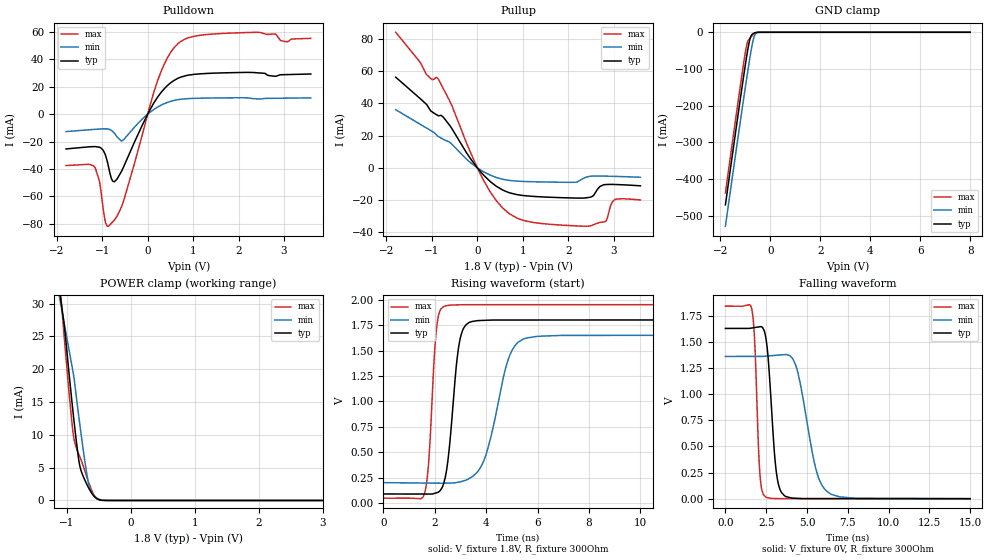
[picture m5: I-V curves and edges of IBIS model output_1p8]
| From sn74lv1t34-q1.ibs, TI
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[Model]   output_1p8
Model_type   Output
Polarity   Non-Inverting
Vmeas = 0.9
Vref = 0.9
Cref = 15pF
Rref = 100000
|   typ   min   max
C_comp   4.947pF   4.835pF   5.043pF
[Voltage Range]   1.8   1.65   1.95
[Temperature Range]   27   125   -40
[Pullup Reference]   1.8   1.65   1.95
[Pulldown Reference]   0   0   0
[Power Clamp Reference]   1.8   1.65   1.95
[GND Clamp Reference]   0   0   0
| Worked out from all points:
|   slope of the pulldown table from 0 to 0.27 V, typ, clamps not added: 18.4 ohm
|   slope of the pullup table from 0 to 0.27 V, typ, clamps not added: 33.4 ohm
|   GND clamp passes 1 mA (typ) near -0.59 V on its own axis
|   POWER clamp passes 1 mA (typ) near -0.60 V on its own axis
|   rising waveform, V_fixture 1.8V, R_fixture 300Ohm: 20-80 % time 371ps typ, 784ps min, 246ps max; typ from 0.092 V to 1.8 V
|   falling waveform, V_fixture 0V, R_fixture 300Ohm: 20-80 % time 430ps typ, 961ps min, 261ps max; typ from 1.63 V to 0 V
[Pulldown]
|   Voltage   I(typ)   I(min)   I(max)
-1.796V   -25.37mA   -12.71mA   -37.49mA
-1.156V   -23.66mA   -11.08mA   -39.01mA
-1.062V   -24.1mA    -10.87mA   -48.82mA
-925mV    -30.32mA   -10.72mA   -79.27mA
-767.5mV  -48.96mA   -12.71mA   -78.42mA
-557.5mV  -40.37mA   -19.33mA   -65.89mA
282.5mV   15.25mA    6.303mA    30mA
576.5mV   24.48mA    9.931mA    48.22mA
839mV     28.01mA    11.17mA    54.92mA
2.414V    30.08mA    11.11mA    59.61mA
3.075V    28.8mA     11.63mA    52.74mA
5.28V     NA         NA         NA
[GND Clamp]
|   Voltage   I(typ)   I(min)   I(max)
-1.796V   -470.7mA   -529mA     -438.3mA
-1.24V    -201.1mA   -262.3mA   -165.8mA
-1.072V   -122.4mA   -183.7mA   -86.98mA
-977.5mV  -79.62mA   -140.4mA   -46.69mA
-904mV    -48.4mA    -107.4mA   -25.58mA
-851.5mV  -29.18mA   -84.47mA   -19.13mA
-799mV    -15.04mA   -62.35mA   -14.79mA
-746.5mV  -7.45mA    -41.87mA   -10.57mA
-673mV    -3.078mA   -18.35mA   -5.616mA
-620.5mV  -1.509mA   -7.62mA    -2.956mA
-568mV    -592.4uA   -2.517mA   -1.156mA
8V        0A         0A         0A
[Pullup]
|   Voltage   I(typ)   I(min)   I(max)
-1.796V   56.2mA     36.07mA    84.03mA
-1.125V   39.5mA     24.8mA     58.02mA
-862mV    32.36mA    19.47mA    55.16mA
-620.5mV  26.8mA     16.08mA    42.2mA
135.5mV   -4.421mA   -2.381mA   -7.688mA
545mV     -13.51mA   -6.947mA   -24.44mA
870.5mV   -16.54mA   -8.182mA   -31.05mA
2.477V    -18.21mA   -5.187mA   -36.01mA
2.824V    -10.32mA   -5.106mA   -33.15mA
2.95V     -10.23mA   -5.193mA   -22.22mA
3.075V    -10.32mA   -5.295mA   -19.28mA
5.28V     NA         NA         NA
[POWER Clamp]
|   Voltage   I(typ)   I(min)   I(max)
-1.796V   83.27mA    70.02mA    99.82mA
-1.114V   32.2mA     31.07mA    33.95mA
-1.04V    26.93mA    27.09mA    25.19mA
-956.5mV  18.76mA    22.59mA    15.78mA
-904mV    13.8mA     19.77mA    10.62mA
-883mV    11.92mA    18.53mA    9.292mA
-799mV    5.487mA    11.92mA    6.762mA
-725.5mV  3.307mA    6.623mA    4.806mA
-662.5mV  2.013mA    2.787mA    2.926mA
-599.5mV  975.7uA    1.075mA    1.342mA
-484mV    84.86uA    158.5uA    58.17uA
8V        0A         0A         0A
[Ramp]
R_load = 300
|   typ   min   max
dV/dt_r   0.978004/5.38655e-10   0.817068/1.18211e-09   1.10595/2.91419e-10
dV/dt_f   1.025/5.79432e-10   0.868241/1.32743e-09   1.13966/3.23116e-10
[Rising Waveform]
V_fixture = 1.8V
V_fixture_min = 1.65V
V_fixture_max = 1.95V
R_fixture = 300Ohm
C_fixture = 0F
|   Time   V(typ)   V(min)   V(max)
0s        91.67mV    202.9mV    50.57mV
1.591ns   91.14mV    199mV      92.11mV
1.753ns   91.08mV    198.6mV    386mV
2.055ns   103.1mV    197.9mV    1.694V
2.354ns   205.2mV    197.2mV    1.933V
2.916ns   1.52V      207.3mV    1.948V
3.317ns   1.773V     240.9mV    1.95V
3.918ns   1.796V     427.4mV    1.95V
5.443ns   1.799V     1.612V     1.95V
15ns      1.8V       1.65V      1.95V
[Falling Waveform]
|Gnd
V_fixture = 0V
V_fixture_min = 0V
V_fixture_max = 0V
R_fixture = 300Ohm
C_fixture = 0F
|   Time   V(typ)   V(min)   V(max)
0s        1.63V      1.362V     1.843V
1.611ns   1.634V     1.362V     1.818V
1.8ns     1.638V     1.362V     1.486V
2.102ns   1.646V     1.362V     268.2mV
2.436ns   1.573V     1.364V     20.52mV
3.113ns   265.1mV    1.373V     1.271mV
3.621ns   28.38mV    1.38V      356.8uV
4.359ns   3.555mV    1.254V     333.9uV
6.187ns   566.5uV    75.08mV    277.5uV
15ns      5.34uV     4.808uV    5.134uV
